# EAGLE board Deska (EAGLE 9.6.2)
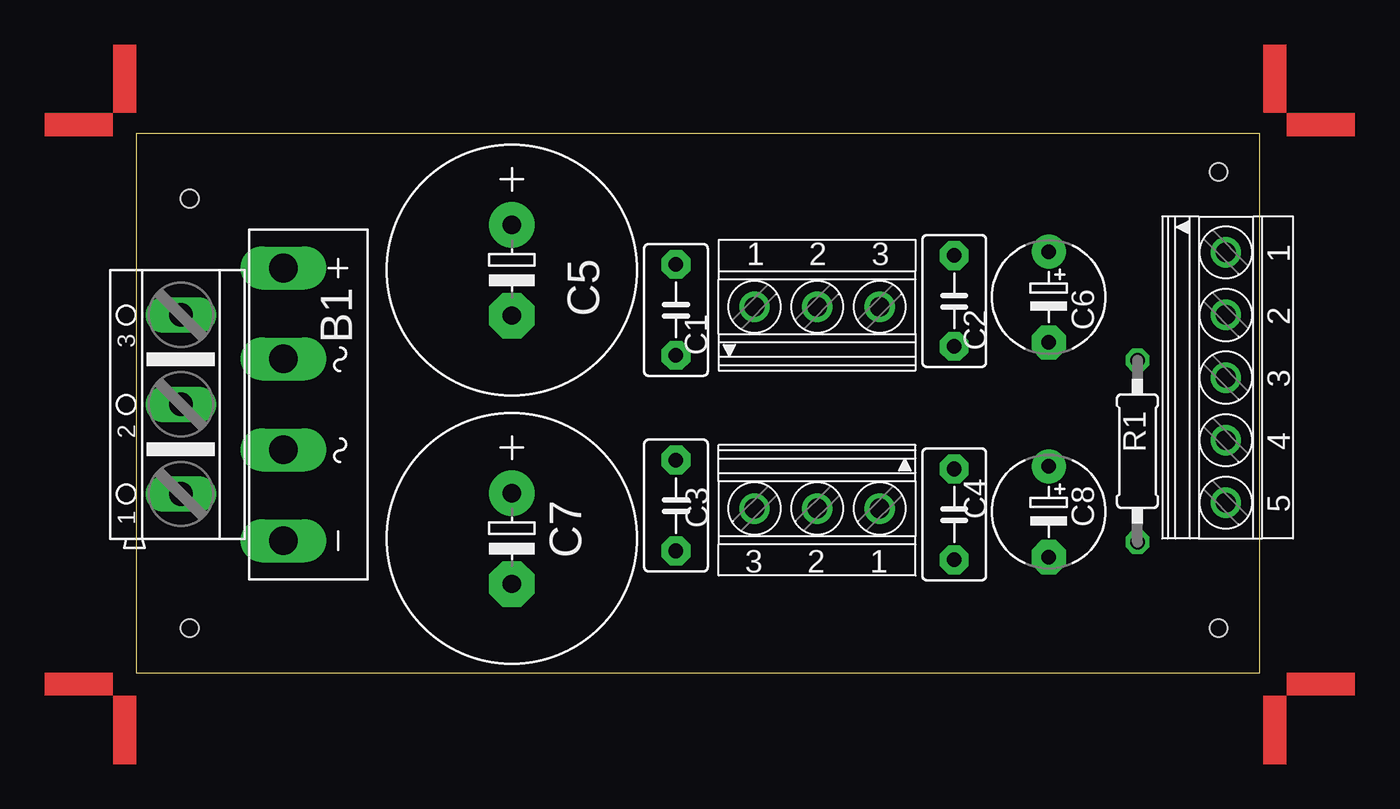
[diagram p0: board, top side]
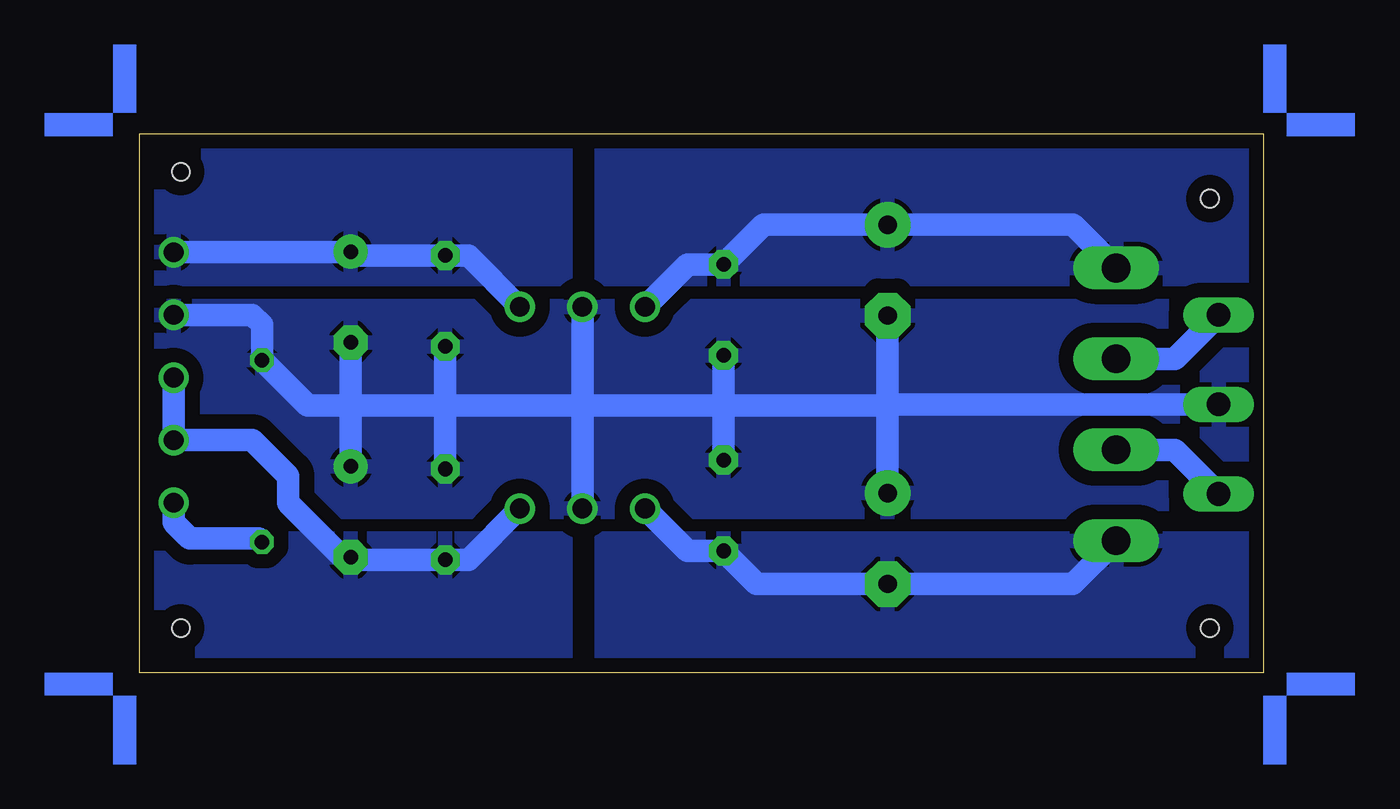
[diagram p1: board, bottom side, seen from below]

Size 62.79 x 30.12 mm. Coordinates in mm from the lower left corner, seen from the top.
Outline: 0,0 62.79,0 62.79,30.12 0,30.12 0,0
Copper layers (1*16): Top 0.035mm / dielectric 1.5mm / Bottom 0.035mm
Design rules "default *": minimum track width 6mil, minimum drill 0.35mm, track to track 6mil, track to pad 6mil, pad to pad 6mil, via to via 6mil, smd to smd 6mil, copper to edge 4mil, drill to drill 6mil, minimum pad ring 10mil, minimum via ring 8mil, stop-mask expansion 4mil, vias tented up to drill 0mil, thermal gap 10mil
Holes 1 mm at 3,26.5 3,2.5 60.5,2.5 60.5,28

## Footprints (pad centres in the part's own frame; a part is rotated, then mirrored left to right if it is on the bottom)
KBL = drill 1.6 long: + -7.62,-1.27; - 7.62,-1.27; AC1 2.54,-1.27; AC2 -2.54,-1.27
C5B3.5 = drill 0.813 pad 1.6 octagon: 1 -2.54,0; 2 2.54,0
E5-13 = drill 1.016 pad 2.54: + -2.54,0 | drill 1.016 pad 2.54 octagon: - 2.54,0
E5-6 = drill 0.813 pad 1.905: + -2.54,0 | drill 0.813 pad 1.905 octagon: - 2.54,0
0207/10 = drill 0.813 octagon: 1 -5.08,0; 2 5.08,0
1751277 = drill 1.1 pad 1.7: 1 -7,-0.1; 2 -3.5,-0.1; 3 0,-0.1; 4 3.5,-0.1; 5 7,-0.1
1751251 = drill 1.1 pad 1.7: 1 -3.5,-0.1; 2 0,-0.1; 3 3.5,-0.1
AK500/3 = drill 1.321 long: 1 -5.004,0; 2 0,0; 3 5.004,0

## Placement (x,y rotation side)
B1  [KBL]  9.5,15 270 top
C1  [C5B3.5]  30.17,20.28 270 top
C2  [C5B3.5]  45.72,20.78 270 top
C3  [C5B3.5]  30.17,9.35 270 top
C4  [C5B3.5]  45.72,8.85 270 top
C5  [E5-13]  21,22.5 270 top
C6  [E5-6]  51,21 270 top
C7  [E5-13]  21,7.5 270 top
C8  [E5-6]  51,9 270 top
R1  [0207/10]  55.96,12.39 90 top
U$1  [ANGLE-SW1-16]  63,30 0 top
U$2  [ANGLE-SW1-16]  0,30 90 top
U$3  [ANGLE-SW1-16]  0,0 180 top
U$4  [ANGLE-SW1-16]  63,0 270 top
X1  1751277  [1751277]  61,16.5 270 top
X3  1751251  [1751251]  38.06,20.55 0 top
X4  1751251  [1751251]  38.06,9.08 180 top
X6  [AK500/3]  2.5,15 90 top

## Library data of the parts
B1 = rectifier
C1-C4 = capacitor-wima
C5-C8 = rcl; SPICEPREFIX: C
R1 = rcl; SPICEPREFIX: R
U$1-U$4 = marks
X1 X3 X4 = con-phoenix-350; OC_FARNELL: unknown; OC_NEWARK: unknown
X6 = con-ptr500; OC_FARNELL: unknown; OC_NEWARK: unknown

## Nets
+12V: C2.1 C6.+ X1.1 X3.3
-12V: C4.2 C8.- X1.3 X1.4 X4.1
GND: C1.2 C2.2 C3.1 C4.1 C5.- C6.- C7.+ C8.+ R1.2 X1.2 X3.2 X4.2 X6.2
N$1: R1.1 X1.5
N$2: B1.- C3.2 C7.- X4.3
N$3: B1.+ C1.1 C5.+ X3.1
N$4: B1.AC2 X6.3
N$5: B1.AC1 X6.1

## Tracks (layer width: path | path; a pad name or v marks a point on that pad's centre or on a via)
+12V
  Bottom 1.27: X3.3 44.43,23.32 C2.1 50.78,23.32 C6.+ | 51.03,23.51 C6.+ | X1.1 51.04,23.5 C6.+
  pour Bottom (isolate 0.813): 63,30 39,30 39,22 63,22
-12V
  Bottom 1.27: X4.1 44.43,6.31 C4.2 50.85,6.31 C8.- 51.46,6.46 54.5,9.5 54.5,11 56.5,13 X1.4 X1.3
  pour Bottom (isolate 0.813): 63,0 63,7.5 39,7.5 39,0
GND
  Bottom 1.27: 21,14.93 30.17,14.93 | 30.17,14.93 38.06,14.93 | 38.06,14.93 45.72,14.93 | 45.72,14.93 51,14.93 | C2.2 45.72,14.93 | C4.1 45.72,14.93 | C1.2 30.17,14.93 | C3.1 30.17,14.93 | X4.2 38.06,14.93 | X3.2 38.06,14.93 | C6.- 51,14.93 | C8.+ 51,14.93 | C5.- 21,14.93 | C7.+ 21,14.93 | 51,14.93 53.42,14.93 R1.2 55.96,19.46 56.5,20 X1.2 | X6.2 20.93,15 21,14.93
  pour Bottom (isolate 0.813): 0,9 63,9 63,20 63,20.5 0,20.5
N$1
  Bottom 1.27: R1.1 56.15,7.5 60,7.5 60.9,8.4 X1.5
N$2
  Bottom 1.27: X4.3 32.19,6.81 C3.2 28.32,4.96 C7.- 10.65,4.96 B1.-
  pour Bottom (isolate 0.813): 0,0 0,7.5 37,7.5 37,0
N$3
  Bottom 1.27: X3.1 32.19,22.82 C1.1 27.95,25.04 C5.+ 10.65,25.04 B1.+
  pour Bottom (isolate 0.813): 0,22 37,22 37,30 0,30
N$4
  Bottom 1.27: X6.3 4.96,17.54 B1.AC2
N$5
  Bottom 1.27: X6.1 4.96,12.46 B1.AC1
